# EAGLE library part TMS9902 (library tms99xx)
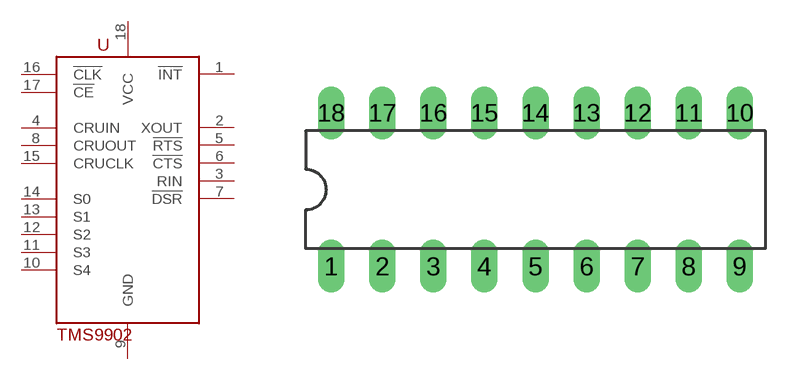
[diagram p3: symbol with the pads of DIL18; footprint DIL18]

Designator prefix -

## TMS9902  [DIL18]
1  !INT  out
2  XOUT  out
3  RIN  in
4  CRUIN  out
5  !RTS  out
6  !CTS  in
7  !DSR  in
8  CRUOUT  in
9  GND  pwr
10  S4  in
11  S3  in
12  S2  in
13  S1  in
14  S0  in
15  CRUCLK  in
16  !CLK  in
17  !CE  in
18  VCC  pwr

## Footprint DIL18 (pad centres in mm)
Dual In Line Package
drill 0.813 long: 1 -10.16,-3.81; 2 -7.62,-3.81; 3 -5.08,-3.81; 4 -2.54,-3.81; 5 0,-3.81; 6 2.54,-3.81; 7 5.08,-3.81; 8 7.62,-3.81; 9 10.16,-3.81; 10 10.16,3.81; 11 7.62,3.81; 12 5.08,3.81; 13 2.54,3.81; 14 0,3.81; 15 -2.54,3.81; 16 -5.08,3.81; 17 -7.62,3.81; 18 -10.16,3.81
